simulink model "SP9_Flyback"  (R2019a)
settings: Solver=VariableStepAuto  StartTime=0  StopTime=0.02  FixedStep=1e-6  RelTol=5e-3
libraries: fl_lib x8, nesl_utility x4, ee_lib x3, powerlib_meascontrol x1

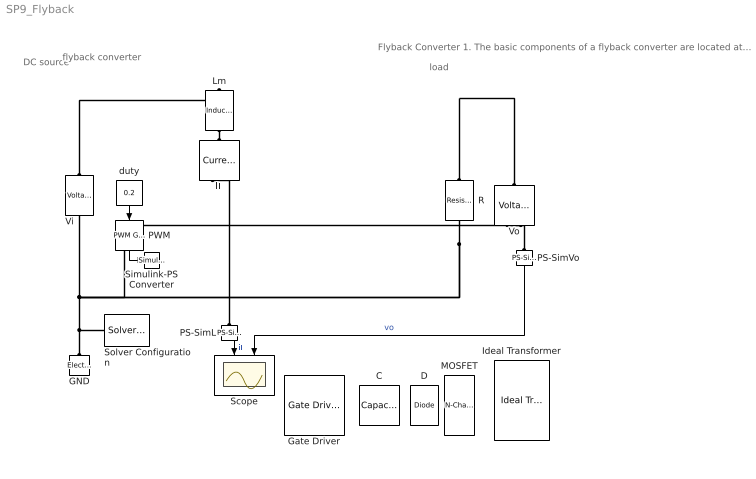
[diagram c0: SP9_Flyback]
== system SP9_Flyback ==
  note: Flyback Converter 1. The basic components of a flyback converter are located at the bottom. 2. Place them in the appropriate positions. Press Ctrl+R to rotate a component. 3. Set the magnetizing inductance to 1 mH, turns ratio to 1:1, and capacitance to 100 uF. (Note the definition of winding ratio in the ideal transformer is N:1, opposite of 1:n learned in class.) C1. Capture the complete circuit diagram. 4. Simulate the circuit. 5. Open the Scope to observe the current and voltage waveforms. C2. Capture the inductor current and output voltage waveforms. Q1. Does this circuit operate in CCM, BCM, or DCM? Q2. What is the output voltage (Vo) and peak-to-peak ripple in steady state? 6. Change the turns ratio to 2:1. C3. Capture the new current and voltage waveforms. Q4. What is the new output voltage (Vo) and peak-to-peak ripple in steady state? Q5. Explain how changing the turns ratio affects the output voltage and ripple. ------------------------------------------------------- 7. Add voltage sensors to measure Vds of the MOSFET and the diode blocking voltage. 8. Copy & paste the scope and two PS-Simulink Converter blocks. 9. Add the two sensor output to the new scope through the PS-Simulink Converter blocks. C4. Capture the new complete circuit diagram. 10. Simulate the circuit. C5. Capture the two new voltage waveforms. Q6. Based on the waveforms, what drain-source voltage rating is required for the MOSFET? Q7. Based on the waveforms, what blocking voltage rating is required for the diode? Q8. Explain why the maximum voltages for each switch is higher than the output and input voltage. _________________________________ Play: Change the inductor or duty ratio so that conduction mode is DCM. Observe how the inductor current and conduction changes in DCM.
  note: load
  note: DC source
  note: flyback converter
  C : fl_lib/Electrical/Electrical Elements/Capacitor  c=1 uF  r=1e-6 Ohm  g=0 1/Ohm  i_specify=off  i_priority=None  i=0 A  i_nominal_specify=off  i_nominal_unit=A  i_nominal_value=1  v_specify=off  v_priority=High  v=20 V  v_nominal_specify=off  v_nominal_unit=V  v_nominal_value=1  vc_specify=off  vc_priority=High  vc=15 V  vc_nominal_specify=off  vc_nominal_unit=V  vc_nominal_value=1
  D : fl_lib/Electrical/Electrical Elements/Diode  Vf=1e-3 V  Ron=1e-3 Ohm  Goff=1e-8 1/Ohm  i_specify=off  i_priority=None  i=0 A  i_nominal_specify=off  i_nominal_unit=A  i_nominal_value=1  v_specify=off  v_priority=None  v=0 V  v_nominal_specify=off  v_nominal_unit=V  v_nominal_value=1
  GND : fl_lib/Electrical/Electrical Elements/Electrical Reference
  Gate Driver : ee_lib/Semiconductors & Converters/Gate Driver  vHigh=15 V  vLow=0 V  parameterization=1  rHigh=2 Ohm  rLow=2 Ohm  tRise=20 ns  tFall=20 ns  cLoad=10 nF  enable_faults=0  t_fault=1 s  fault_type=1  uHighValue=0.7  uLowValue=0.3  tHigh=50 ns  tLow=50 ns  ZonTime_specify=off  ZonTime_priority=None  ZonTime=0 s  ZoffTime_specify=off  ZoffTime_priority=None  ZoffTime=0 s  uHigh=2.0 V  uLow=0.8 V
  Ideal Transformer : fl_lib/Electrical/Electrical Elements/Ideal Transformer  n=10  i1_specify=off  i1_priority=None  i1=0 A  i1_nominal_specify=off  i1_nominal_unit=A  i1_nominal_value=1  v1_specify=off  v1_priority=None  v1=0 V  v1_nominal_specify=off  v1_nominal_unit=V  v1_nominal_value=1  i2_specify=off  i2_priority=None  i2=0 A  i2_nominal_specify=off  i2_nominal_unit=A  i2_nominal_value=1  v2_specify=off  v2_priority=None  v2=0 V  v2_nominal_specify=off  v2_nominal_unit=V  v2_nominal_value=1
  Lm : fl_lib/Electrical/Electrical Elements/Inductor  l=10 uH  r=0 Ohm  g=1e-9 1/Ohm  i_specify=off  i_priority=None  i=0.291 A  i_nominal_specify=off  i_nominal_unit=A  i_nominal_value=1  v_specify=off  v_priority=None  v=0 V  v_nominal_specify=off  v_nominal_unit=V  v_nominal_value=1  i_L_specify=off  i_L_priority=High  i_L=0.291 A  i_L_nominal_specify=off  i_L_nominal_unit=A  i_L_nominal_value=1
  MOSFET : ee_lib/Semiconductors & Converters/N-Channel MOSFET  parameterization=1  prmDatasheet=1  prmEquCoeff=1  Beta=5.0 A/V^2  Rds=0.025 Ohm  Id=6.0 A  Vgs=10 V  Vth=1.7 V  lam=0 1/V  Tmeas=25 degC  RS=0.0001 Ohm  RD=0.01 Ohm  C_param=1  C_GS=270 pF  C_GD=80 pF  C_DS=0 pF  C_iss=350 pF  C_rss=80 pF  C_oss=0 pF  C_GS_vec=[270, 300, 290, 280, 295, 255] pF  C_GD_vec=[450, 400, 300, 190, 95, 55] pF  C_DS_vec=[450, 410, 390, 230, 175, 115] pF  C_iss_vec=[720, 700, 590, 470, 390, 310] pF  C_rss_vec=[450, 400, 300, 190, 95, 55] pF  C_oss_vec=[900, 810, 690, 420, 270, 170] pF  C_Vds_vec=[.1, .3, 1, 3, 10, 30] V  V_GS_for_cap_data=0 V  charge_linearity_param=1  C_OX=200 pF  V_C_OX=-0.5 V  IsDiode=0 A  Vbi=0.6 V  n=1  Cj0Diode=0 pF  TT=50e-9 s  dVth_dT=-6 mV/K  Rds_T2=0.037 Ohm  Tmeas2=125 degC  BEXDatasheet=-1.5  BEXEquCoeff=-1.5  etaisDatasheet=3  etaisEquCoeff=3  TdeviceDatasheet=25 degC  TdeviceEquCoeff=25 degC  Rth=[1, 10] K/W  thermal_mass_parameterization=1  thermal_mass=[1, 1] J/K  thermal_time_constant=[1, 10] s  thermal_mass_initial_temperatures=[25, 25] degC  betaref=18 A/V^2  Vfbref=-1.1 V  gamma=3.5 V^0.50000  phib2ref=1 V  thesatref=0.4 1/V  alpha=0  Vp=5e-2 V  thesrref=0 1/V  m=8  Tref=25 degC  Cox=1500 pF  Cgso=100 pF  Cgdo=14 pF  Rsref=2e-3 Ohm  Rdref=0.17 Ohm  Rgref=8.4 Ohm  Isref=5.2e-13 A  Cj0=480 pF  Tprm=1  etabet=1.3  Stvfb=5e-4 V/K  Stphib=-8.5e-4 V/K  etasat=1.04  etasr=0.65  etar=0.95  etais=3  Tsim=25 degC  T0=[25, 25] degC
  PS-SimL : nesl_utility/PS-Simulink Converter  PhysicalDomain=network_engine_domain  SubClassName=ps_output  LeftPortType=input  RightPortType=output  PseudoPeriodic=off  Frequencies=[]  Unit=1  AffineConversion=off
  PS-SimVo : nesl_utility/PS-Simulink Converter  PhysicalDomain=network_engine_domain  SubClassName=ps_output  LeftPortType=input  RightPortType=output  PseudoPeriodic=off  Frequencies=[]  Unit=1  AffineConversion=off
  PWM : powerlib_meascontrol/Pulse & Signal Generators/PWM Generator (DC-DC)  Fsw=10000  Ts=0
  R : fl_lib/Electrical/Electrical Elements/Resistor  R=1 Ohm  i_specify=off  i_priority=None  i=0 A  i_nominal_specify=off  i_nominal_unit=A  i_nominal_value=1  v_specify=off  v_priority=None  v=0 V  v_nominal_specify=off  v_nominal_unit=V  v_nominal_value=1
  Scope : Scope  NumInputPorts=2
  Simulink-PS Converter : nesl_utility/Simulink-PS Converter  PhysicalDomain=network_engine_domain  SubClassName=ps_input  LeftPortType=input  RightPortType=output  PseudoPeriodic=off  Frequencies=[]  NoiseDistribution=none  NoiseParameters=[]  Unit=1  AffineConversion=off  FilteringAndDerivatives=provide  SimscapeFilterOrder=1  InputFilterTimeConstant=0.001  UdotUserProvided=0
  Solver Configuration : nesl_utility/Solver Configuration  PhysicalDomain=network_engine_domain  SubClassName=solver  LeftPortType=input  RightPortType=generic  Tones=[]  Harmonics=[]  SimulateNoise=off  Profile=off  UseLocalSampling=off  EnableSwitchedLinearOptims=on  FrequencyDomain=off  UseCCode=off  RelTol=0.001  AbsTol=1e-06  MinStep=1e-09  ToWorkspace=off  RevertToSquareIcSolve=off  NumHomotopyIterations=100  PhasorMode=off  PhasorModeNumHarmonics=1  DoDC=off  ResidualTolerance=1e-09  UseLocalSolver=off  LocalSolverChoice=NE_BACKWARD_EULER_ADVANCER  LocalSolverSampleTime=0.001  DoFixedCost=off  MaxNonlinIter=3  MaxModeIter=2  LinearAlgebra=auto  EquationFormulation=NE_TIME_EF  DelaysMemoryBudget=1024  AutomaticFiltering=on  FilteringTimeConstant=0.001  PartitionStorageMethod=AS_NEEDED  PartitionMemoryBudget=1024  PartitionMethod=ROBUST
  Vi : ee_lib/Sources/Voltage Source  dc_voltage=10 V  ac_voltage=0 V  ac_shift=0 rad  ac_frequency=60 Hz  noise_mode=0  PSD=0 V^2/Hz  repeatability=1  auto_seed=3646982598  user_seed=0  sample_time=1e-3 s  i_specify=off  i_priority=None  i=0 A  i_nominal_specify=off  i_nominal_unit=A  i_nominal_value=1  v_specify=off  v_priority=None  v=0 V  v_nominal_specify=off  v_nominal_unit=V  v_nominal_value=1
  Vo : fl_lib/Electrical/Electrical Sensors/Voltage Sensor
  duty : Constant  Value=0.2
  iL : fl_lib/Electrical/Electrical Sensors/Current Sensor
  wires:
  PWM/1 -> Simulink-PS Converter/1
  duty/1 -> PWM/1
  PS-SimL/1 -> Scope/1  "iL"
  PS-SimVo/1 -> Scope/2  "vo"
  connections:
  PS-SimVo/LConn1 -- Vo/RConn1
  R/LConn1 -- Vo/LConn1
  PS-SimL/LConn1 -- iL/RConn1
  Vi/LConn1 -- Lm/LConn1
  R/RConn1 -- Vo/RConn2 -- Vi/RConn1 -- Solver Configuration/RConn1 -- GND/LConn1
  iL/LConn1 -- Lm/RConn1
